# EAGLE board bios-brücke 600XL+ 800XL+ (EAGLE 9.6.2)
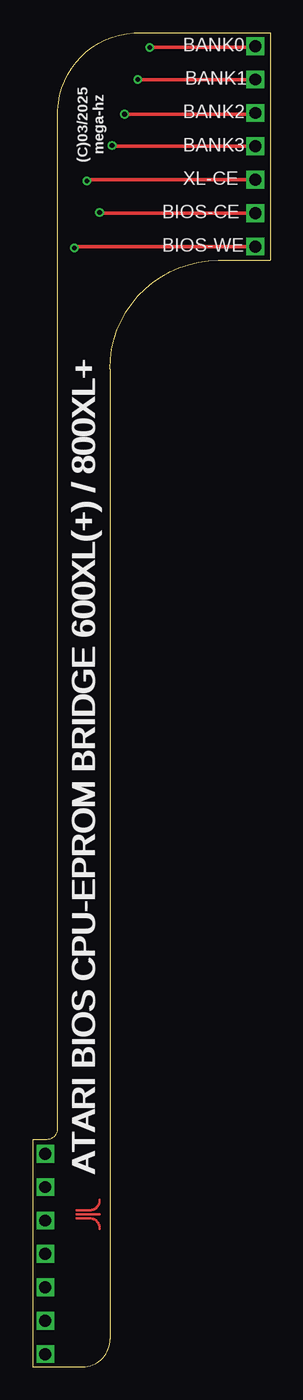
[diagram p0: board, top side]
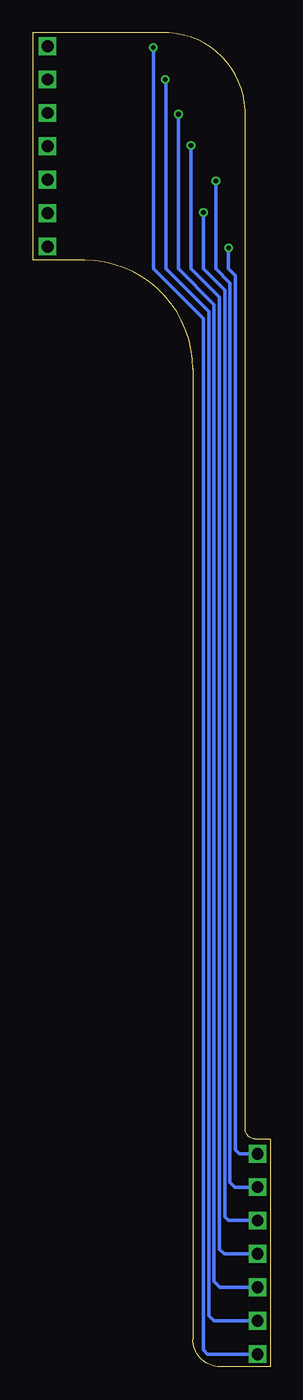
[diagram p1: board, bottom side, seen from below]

Size 18.07 x 101.44 mm. Coordinates in mm from the lower left corner, seen from the top.
Outline: 0,17.3 0,0 3.81,0 arc90 5.87,2.06 5.87,75.88 arc-90 14.13,84.14 18.07,84.14 18.07,101.44 8.25,101.44 arc90 1.91,95.57 1.91,18.1 arc-90 1.11,17.3 0,17.3
Copper layers (1+2*15+16): Top 0.035mm / dielectric 1.5mm / Route2 0.035mm / dielectric 0.15mm / Route15 0.035mm / dielectric 0.2mm / Bottom 0.035mm
Design rules "ITead_rule *": minimum track width 6mil, minimum drill 12mil, track to track 6mil, track to pad 6mil, pad to pad 6mil, via to via 6mil, smd to smd 0mil, copper to edge 10mil, drill to drill 10mil, minimum pad ring 10mil, minimum via ring 6mil, stop-mask expansion 2mil, vias tented up to drill 100mil, thermal gap 10mil

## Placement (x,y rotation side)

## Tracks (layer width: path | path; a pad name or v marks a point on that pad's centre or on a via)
B0  (via drill 0.35, 0.9)
  Top 0.254: v16.95,100.43 16.85,100.33 v8.89,100.33
  Bottom 0.254: v0.95,0.95 4.76,0.95 5.08,1.27 5.08,79.69 8.89,83.5 v8.89,100.33
B1  (via drill 0.35, 0.9)
  Top 0.254: v16.95,97.89 v7.99,97.89
  Bottom 0.254: v0.95,3.49 4.29,3.49 4.67,3.88 4.67,80.24 7.94,83.5 7.94,97.84 v7.99,97.89
B2  (via drill 0.35, 0.9)
  Top 0.254: v16.95,95.35 16.85,95.25 v6.99,95.25
  Bottom 0.254: v0.95,6.03 3.81,6.03 4.27,6.49 4.27,80.78 6.99,83.5 v6.99,95.25
B3  (via drill 0.35, 0.9)
  Top 0.254: v16.95,92.81 6.09,92.81 v6.03,92.87
  Bottom 0.254: v0.95,8.57 3.49,8.57 3.86,8.94 3.86,81.33 6.03,83.5 v6.03,92.87
BIOS  (via drill 0.35, 0.9)
  Top 0.254: v16.95,87.73 5.14,87.73 v5.08,87.79
  Bottom 0.254: v0.95,11.11 3.17,11.11 3.45,11.39 3.45,81.88 5.08,83.5 v5.08,87.79
EE_RW  (via drill 0.35, 0.9)
  Top 0.254: v16.95,85.19 3.28,85.19 v3.17,85.09
  Bottom 0.254: v0.95,16.19 2.36,16.19 2.64,16.48 2.64,82.97 3.17,83.5 v3.17,85.09
N$1
  Top 0.2: 3.33,11.91 4.45,11.91
N$2
  Top 0.2: 4.45,11.91 arc90 5.08,12.7
N$3
  Top 0.2: 3.33,11.59 5.08,11.59
N$4
  Top 0.2: 3.33,11.27 4.45,11.27
N$5
  Top 0.2: 4.45,11.27 arc-90 5.08,10.48
XLOS  (via drill 0.35, 0.9)
  Top 0.254: v16.95,90.27 4.23,90.27 v4.13,90.17
  Bottom 0.254: v0.95,13.65 2.7,13.65 3.05,14 3.05,82.42 4.13,83.5 v4.13,90.17

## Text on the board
tPlace: BANK0 | BANK1 | BANK2 | (C)03/2025 / mega-hz | BANK3 | XL-CE | BIOS-CE | BIOS-WE | ATARI BIOS CPU-EPROM BRIDGE 600XL(+) / 800XL+ | ATARI BIOS CPU-EPROM BRIDGE 600XL(+) / 800XL+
